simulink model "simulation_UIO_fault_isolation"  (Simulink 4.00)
settings: Solver=VariableStepDiscrete  StartTime=0.0  StopTime=ts  RelTol=1e-3
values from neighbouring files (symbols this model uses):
  A = [0.9944 -0.1203 -0.4302    [UIO_fault_isolation.m]
  Auio1 = F1    [UIO_fault_isolation.m]
  Auio2 = F2    [UIO_fault_isolation.m]
  B = [1 0    [UIO_fault_isolation.m]
  Buio1 = [T1*B K1]    [UIO_fault_isolation.m]
  Buio2 = [T2*B K2]    [UIO_fault_isolation.m]
  C = eye(3)    [UIO_fault_isolation.m]
  Cuio1 = C    [UIO_fault_isolation.m]
  Cuio2 = C    [UIO_fault_isolation.m]
  D = zeros(3,3)    [UIO_fault_isolation.m]
  Duio1 = [zeros(3,2) H1]    [UIO_fault_isolation.m]
  Duio2 = [zeros(3,2) H2]    [UIO_fault_isolation.m]
  Tc = 0.1    [UIO_fault_isolation.m]
  x0 = [0.01 0.02 0.03]    [UIO_fault_isolation.m]

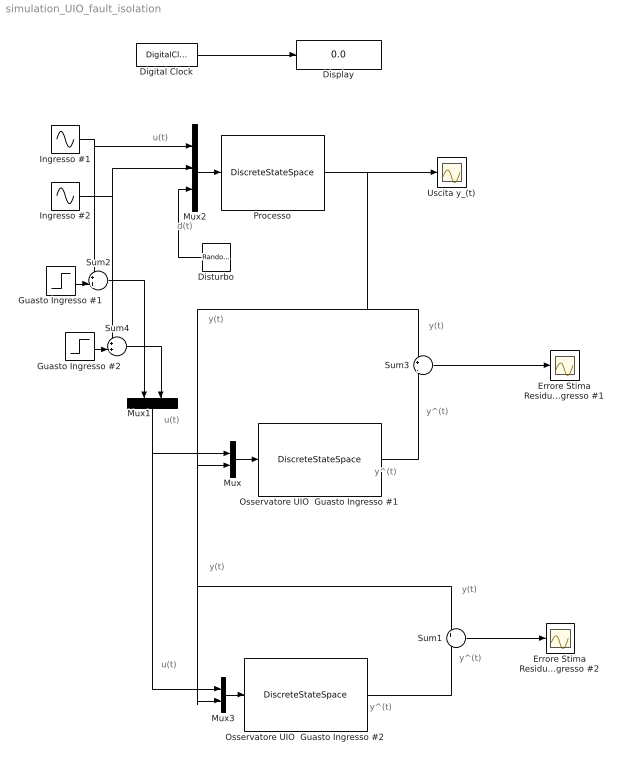
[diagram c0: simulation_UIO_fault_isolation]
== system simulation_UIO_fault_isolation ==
  note: u(t)
  note: y^(t)
  note: y(t)
  note: y^(t)
  note: y^(t)
  note: y^(t)
  note: y(t)
  note: d(t)
  note: u(t)
  note: u(t)
  note: y(t)
  note: y(t)
  Digital Clock : DigitalClock  SampleTime=Tc
  Display : Display
  Disturbo : RandomNumber  Orientation=left  Mean=0  Variance=0.05  Seed=0  SampleTime=Tc
  Errore Stima Residuo Ingresso #1 : Scope
  Errore Stima Residuo Ingresso #2 : Scope
  Guasto Ingresso #1 : Step  Time=25  Before=0  After=0  SampleTime=0
  Guasto Ingresso #2 : Step  Time=25  Before=0  After=1  SampleTime=0
  Ingresso #1 : Sin  SineType=Time-based  Amplitude=1  Bias=0  Frequency=1  Phase=0  Samples=10  SampleTime=Tc
  Ingresso #2 : Sin  SineType=Time-based  Amplitude=1  Bias=0  Frequency=1  Phase=pi/2  Samples=10  SampleTime=Tc
  Mux : Mux  Inputs=2
  Mux1 : Mux  Orientation=down  Inputs=2
  Mux2 : Mux  Inputs=3
  Mux3 : Mux  Inputs=2
  Osservatore UIO  Guasto Ingresso #1 : DiscreteStateSpace  A=Auio1  B=Buio1  C=Cuio1  D=Duio1  X0=0  SampleTime=Tc  Realization=auto
  Osservatore UIO  Guasto Ingresso #2 : DiscreteStateSpace  A=Auio2  B=Buio2  C=Cuio2  D=Duio2  X0=0  SampleTime=Tc  Realization=auto
  Processo : DiscreteStateSpace  A=A  B=[B E]  C=C  D=D  X0=x0  SampleTime=Tc  Realization=auto
  Sum1 : Sum  Inputs=+|-  SaturateOnIntegerOverflow=on
  Sum2 : Sum  Inputs=++|  SaturateOnIntegerOverflow=on
  Sum3 : Sum  Inputs=+|-  SaturateOnIntegerOverflow=on
  Sum4 : Sum  Inputs=++|  SaturateOnIntegerOverflow=on
  Uscita y_(t) : Scope
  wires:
  Digital Clock/1 -> Display/1
  Mux2/1 -> Processo/1
  Ingresso #1/1 -> Mux2/1, Sum2/1
  Processo/1 -> Sum3/1, Mux/2, Mux3/2, Sum1/1, Uscita y_(t)/1
  Mux/1 -> Osservatore UIO  Guasto Ingresso #1/1
  Osservatore UIO  Guasto Ingresso #1/1 -> Sum3/2
  Sum3/1 -> Errore Stima Residuo Ingresso #1/1
  Mux3/1 -> Osservatore UIO  Guasto Ingresso #2/1
  Osservatore UIO  Guasto Ingresso #2/1 -> Sum1/2
  Sum1/1 -> Errore Stima Residuo Ingresso #2/1
  Disturbo/1 -> Mux2/3
  Guasto Ingresso #1/1 -> Sum2/2
  Ingresso #2/1 -> Mux2/2, Sum4/1
  Guasto Ingresso #2/1 -> Sum4/2
  Mux1/1 -> Mux/1, Mux3/1
  Sum4/1 -> Mux1/2
  Sum2/1 -> Mux1/1
